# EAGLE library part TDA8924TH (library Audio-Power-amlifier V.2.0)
The TDA8924 is a high efficiency class-D audio power amplifier with very low dissipation. The typical output power is 2 ´ 120 W. The device comes in a HSOP24 power package with a small internal heatsink. Depending on supply voltage and load conditions a very small or even no external heatsink is required. The amplifier operates over a wide supply voltage range from ±12.5 V to ±30 V and consumes a very low quiescent current.
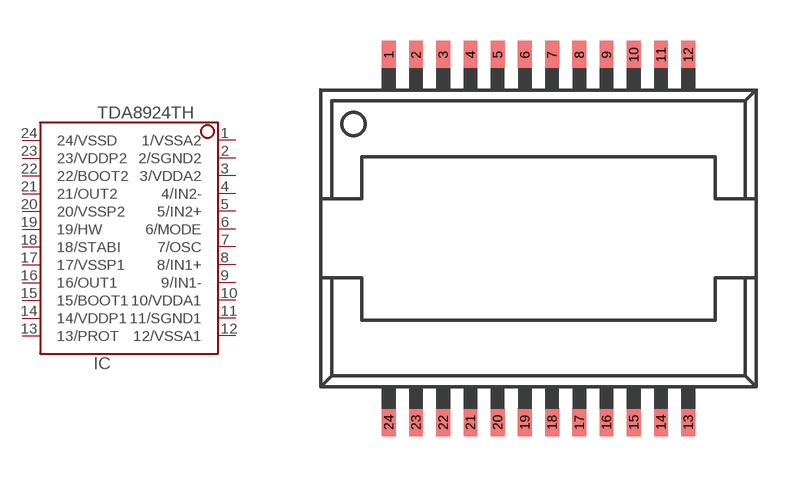
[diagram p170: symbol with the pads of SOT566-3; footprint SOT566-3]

Designator prefix IC

## TDA8924TH  [SOT566-3]
1  1/VSSA2  pwr
2  2/SGND2  pwr
3  3/VDDA2  pwr
4  4/IN2-  in
5  5/IN2+  in
6  6/MODE  in
7  7/OSC  in
8  8/IN1+  in
9  9/IN1-  in
10  10/VDDA1  pwr
11  11/SGND1  pwr
12  12/VSSA1  pwr
13  13/PROT
14  14/VDDP1  pwr
15  15/BOOT1
16  16/OUT1  out
17  17/VSSP1  pwr
18  18/STABI
19  19/HW
20  20/VSSP2  pwr
21  21/OUT2  out
22  22/BOOT2
23  23/VDDP2  pwr
24  24/VSSD  pwr

## Footprint SOT566-3 (pad centres in mm)
smd 0.508 x 1.016: 1 -5.5,6.75; 2 -4.5,6.75; 3 -3.5,6.75; 4 -2.5,6.75; 5 -1.5,6.75; 6 -0.5,6.75; 7 0.5,6.75; 8 1.5,6.75; 9 2.5,6.75; 10 3.5,6.75; 11 4.5,6.75; 12 5.5,6.75; 13 5.5,-6.75; 14 4.5,-6.75; 15 3.5,-6.75; 16 2.5,-6.75; 17 1.5,-6.75; 18 0.5,-6.75; 19 -0.5,-6.75; 20 -1.5,-6.75; 21 -2.5,-6.75; 22 -3.5,-6.75; 23 -4.5,-6.75; 24 -5.5,-6.75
